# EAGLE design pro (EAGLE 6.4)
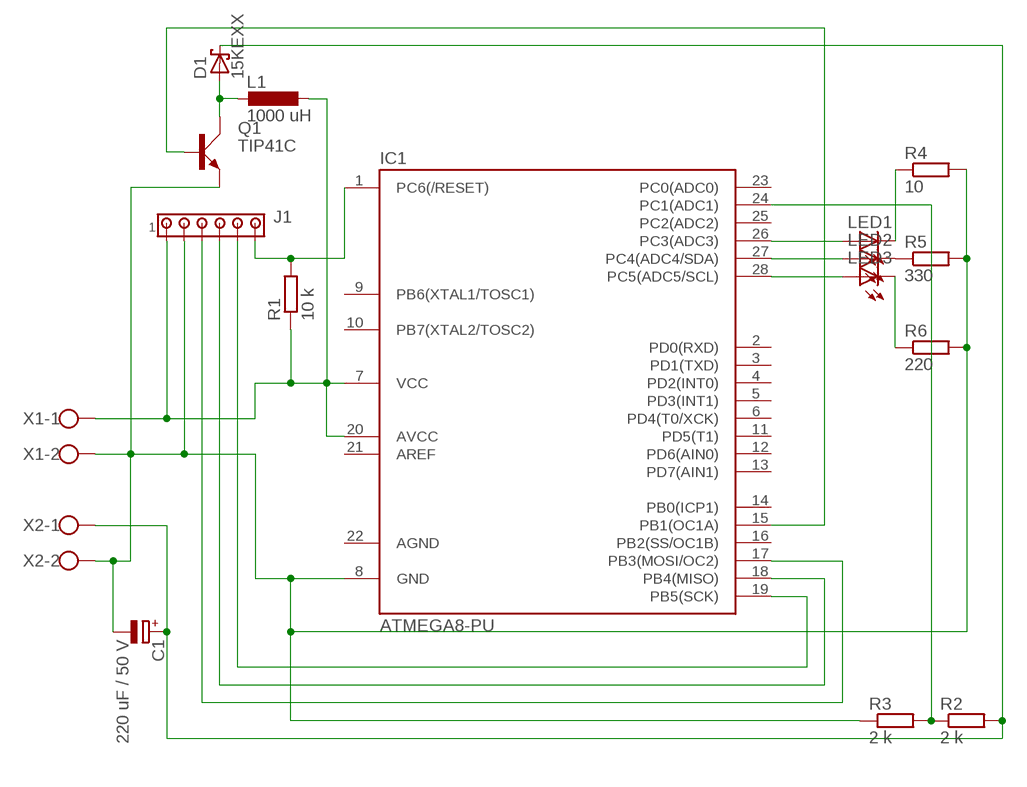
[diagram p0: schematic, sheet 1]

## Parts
C1  220 uF / 50 V  CPOL-EUE3.5-10  [E3,5-10]
D1  15KEXX  [CB429-17]
IC1  ATMEGA8-PU  [DIL28-3]
J1  MTA06-100  [10X06MTA]
L1  1000 uH  L-EUTJ5-U1  [TJ5-U1]
LED1  LED5MM  [LED5MM]
LED2  LED5MM  [LED5MM]
LED3  LED5MM  [LED5MM]
Q1  TIP41C  [TO220AV]
R1  10 k  R-EU_0204/7  [0204/7]
R2  2 k  R-EU_0204/7  [0204/7]
R3  2 k  R-EU_0204/7  [0204/7]
R4  10  R-EU_0204/7  [0204/7]
R5  330  R-EU_0204/7  [0204/7]
R6  220  R-EU_0204/7  [0204/7]
X1  W237-102  [W237-102]
X2  W237-102  [W237-102]

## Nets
N$1: IC1.7(VCC) IC1.20(AVCC) J1.6 L1.1 R1.1 X1.1
N$2: IC1.26(PC3(ADC3)) LED1.A
N$3: IC1.19(PB5(SCK)) J1.2
N$4: IC1.1(PC6(/RESET)) J1.1 R1.2
N$5: IC1.18(PB4(MISO)) J1.3
N$6: IC1.17(PB3(MOSI/OC2)) J1.4
N$7: LED1.K(C) R4.1
N$8: IC1.24(PC1(ADC1)) R2.1 R3.2
N$9: C1.+ D1.C R2.2 X2.1
N$10: D1.A L1.2 Q1.C
N$11: IC1.15(PB1(OC1A)) Q1.B
N$12: IC1.27(PC4(ADC4/SDA)) LED2.A
N$13: LED3.K(C) R6.1
N$14: LED2.K(C) R5.1
N$15: C1.- IC1.8(GND) J1.5 Q1.E R3.1 R4.2 R5.2 R6.2 X1.2 X2.2
N$16: IC1.28(PC5(ADC5/SCL)) LED3.A
Unconnected: IC1.2(PD0(RXD)) IC1.3(PD1(TXD)) IC1.4(PD2(INT0)) IC1.5(PD3(INT1)) IC1.6(PD4(T0/XCK)) IC1.9(PB6(XTAL1/TOSC1)) IC1.10(PB7(XTAL2/TOSC2)) IC1.11(PD5(T1)) IC1.12(PD6(AIN0)) IC1.13(PD7(AIN1)) IC1.14(PB0(ICP1)) IC1.16(PB2(SS/OC1B)) IC1.21(AREF) IC1.23(PC0(ADC0)) IC1.25(PC2(ADC2))

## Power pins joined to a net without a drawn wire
AGND: IC1.22(AGND)

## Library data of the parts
C1 = rcl:CPOL-EU: POLARIZED CAPACITOR, European symbol
D1 = diode:15KEXX: DIODE
IC1 = atmega8:ATMEGA8-PU
J1 = con-amp:MTA06-100: AMP connector
L1 = rcl:L-EU: INDUCTOR, European symbol
LED1-LED3 = led:LED: LED
Q1 = transistor-power:TIP41C: NPN TRANSISTOR
R1-R6 = resistor:R-EU_: RESISTOR, European symbol
X1 X2 = con-wago-500:W237-102: WAGO SCREW CLAMP; MPN: 237-102; OC_FARNELL: unknown; OC_NEWARK: 70K9898

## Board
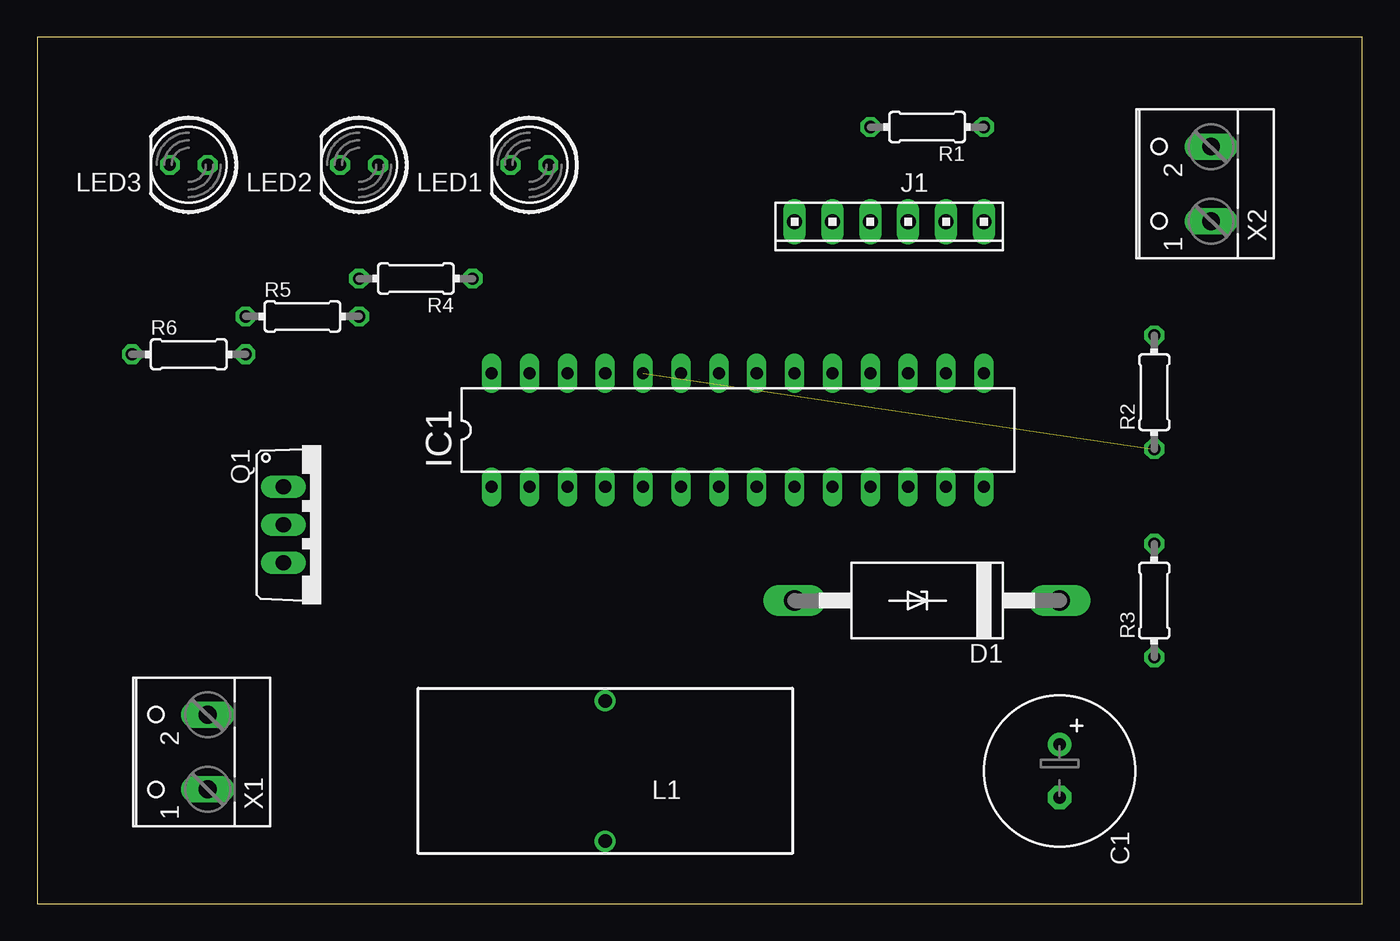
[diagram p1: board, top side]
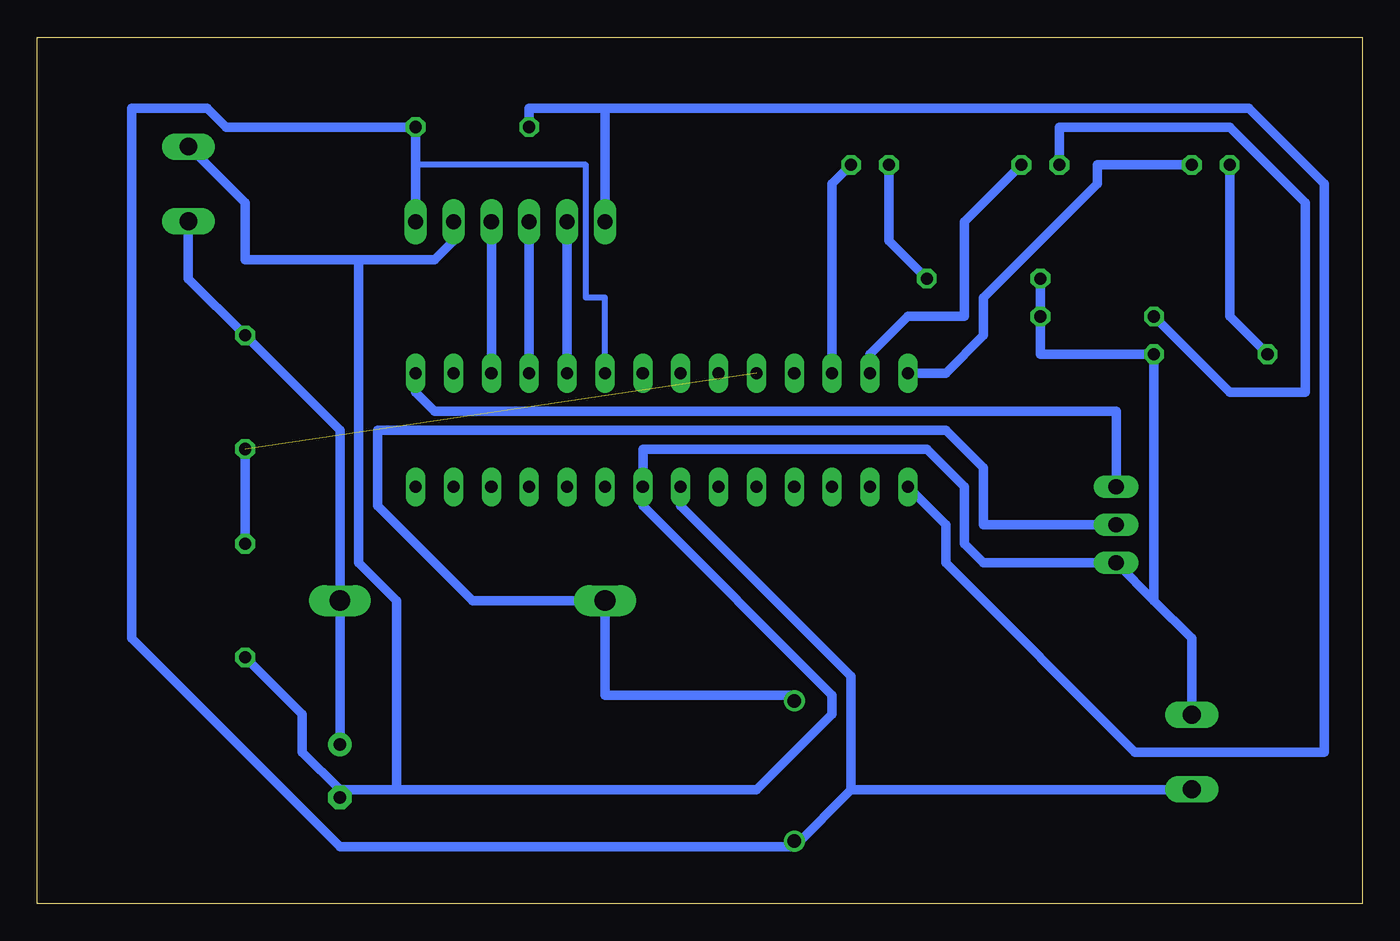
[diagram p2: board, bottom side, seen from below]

Size 88.88 x 58.09 mm. Coordinates in mm from the lower left corner, seen from the top.
Outline: 0,0 88.88,0 88.88,58.09 0,58.09 0,0
Copper layers (1*16): Top 0.035mm / dielectric 1.5mm / Bottom 0.035mm
Design rules "default *": minimum track width 25mil, minimum drill 24mil, track to track 22mil, track to pad 22mil, pad to pad 8mil, via to via 8mil, smd to smd 8mil, copper to edge 40mil, drill to drill 8mil, minimum pad ring 10mil, minimum via ring 8mil, stop-mask expansion 4mil, vias tented up to drill 0mil, thermal gap 10mil

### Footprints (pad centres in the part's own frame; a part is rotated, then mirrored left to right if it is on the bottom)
E3,5-10 = drill 0.813 pad 1.6: + -1.778,0 | drill 0.813 pad 1.6 octagon: - 1.778,0
CB429-17 = drill 1.397 long: A 8.89,0; C -8.89,0
DIL28-3 = drill 0.813 long: 1 -16.51,-3.81; 2 -13.97,-3.81; 3 -11.43,-3.81; 4 -8.89,-3.81; 5 -6.35,-3.81; 6 -3.81,-3.81; 7 -1.27,-3.81; 8 1.27,-3.81; 9 3.81,-3.81; 10 6.35,-3.81; 11 8.89,-3.81; 12 11.43,-3.81; 13 13.97,-3.81; 14 16.51,-3.81; 15 16.51,3.81; 16 13.97,3.81; 17 11.43,3.81; 18 8.89,3.81; 19 6.35,3.81; 20 3.81,3.81; 21 1.27,3.81; 22 -1.27,3.81; 23 -3.81,3.81; 24 -6.35,3.81; 25 -8.89,3.81; 26 -11.43,3.81; 27 -13.97,3.81; 28 -16.51,3.81
10X06MTA = drill 1.016 long: 1 6.35,0; 2 3.81,0; 3 1.27,0; 4 -1.27,0; 5 -3.81,0; 6 -6.35,0
TJ5-U1 = drill 0.9: 1 -4.7,0; 2 4.7,0
LED5MM = drill 0.813 octagon: A -1.27,0; K 1.27,0
TO220AV = drill 1.016 long: B -2.54,-2.54; C 0,-2.54; E 2.54,-2.54
0204/7 = drill 0.813 octagon: 1 -3.81,0; 2 3.81,0
W237-102 = drill 1.194 long: 1 -2.5,-1.27; 2 2.5,-1.27

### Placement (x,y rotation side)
C1  68.58,8.89 270 top
D1  59.69,20.32 180 top
IC1  46.99,31.75 0 top
J1  57.15,45.72 180 top
L1  38.1,8.89 90 top
LED1  33.02,49.53 180 top
LED2  21.59,49.53 180 top
LED3  10.16,49.53 180 top
Q1  19.05,25.4 270 top
R1  59.69,52.07 180 top
R2  74.93,34.29 90 top
R3  74.93,20.32 90 top
R4  25.4,41.91 180 top
R5  17.78,39.37 0 top
R6  10.16,36.83 0 top
X1  10.16,10.16 90 top
X2  77.47,48.26 90 top

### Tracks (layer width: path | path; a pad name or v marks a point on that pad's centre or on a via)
N$1
  Bottom 0.406: IC1.20 50.8,40.64 52.07,40.64 52.07,49.53 63.5,49.53
  Bottom 0.635: J1.6 63.5,49.53 R1.1 76.2,52.07 77.47,53.34 82.55,53.34 82.55,17.78 68.58,3.81 38.1,3.81 | IC1.7 45.72,26.67 34.29,15.24 34.29,7.62 | 38.1,3.81 34.29,7.62 | 34.29,7.62 11.43,7.62 X1.1 | 38.1,3.81 L1.1
N$2
  Bottom 0.635: IC1.26 35.56,48.26 LED1.A
N$3
  Bottom 0.635: J1.2 IC1.19
N$4
  Bottom 0.635: IC1.1 27.94,25.4 27.94,22.86 15.24,10.16 2.54,10.16 2.54,48.26 7.62,53.34 50.8,53.34 | 50.8,53.34 55.88,53.34 R1.2 | 50.8,53.34 J1.1
N$5
  Bottom 0.635: J1.3 IC1.18
N$6
  Bottom 0.635: J1.4 IC1.17
N$7
  Bottom 0.635: R4.1 31.75,44.45 LED1.K
N$8  (1 unrouted)
  Bottom 0.635: R2.1 R3.2
N$9
  Bottom 0.635: X2.1 78.74,41.91 R2.2 68.58,31.75 D1.C C1.+
N$10
  Bottom 0.635: L1.2 38.1,13.97 50.8,13.97 D1.A 59.69,20.32 66.04,26.67 66.04,31.75 27.94,31.75 25.4,29.21 25.4,25.4 Q1.C
N$11
  Bottom 0.635: IC1.15 63.5,34.29 62.23,33.02 16.51,33.02 Q1.B
N$12
  Bottom 0.635: IC1.27 33.02,36.83 30.48,39.37 26.67,39.37 26.67,45.72 LED2.A
N$13
  Bottom 0.635: R6.1 8.89,39.37 LED3.K
N$14
  Bottom 0.635: R5.1 8.89,34.29 3.81,34.29 3.81,46.99 8.89,52.07 20.32,52.07 LED2.K
N$15
  Bottom 0.635: R4.2 R5.2 21.59,36.83 R6.2 13.97,20.32 | 13.97,20.32 11.43,17.78 X1.2 | 13.97,20.32 Q1.E 25.4,22.86 26.67,24.13 26.67,27.94 29.21,30.48 48.26,30.48 IC1.8 48.26,26.67 35.56,13.97 35.56,12.7 40.64,7.62 64.77,7.62 | J1.5 60.96,44.45 62.23,43.18 67.31,43.18 | 67.31,43.18 74.93,43.18 74.93,46.99 78.74,50.8 X2.2 | 68.58,7.62 64.77,7.62 | R3.1 71.12,12.7 71.12,10.16 68.58,7.62 | 68.58,7.62 C1.- | 67.31,43.18 67.31,22.86 64.77,20.32 64.77,7.62
N$16
  Bottom 0.635: LED3.A 17.78,49.53 17.78,48.26 25.4,40.64 25.4,38.1 27.94,35.56 IC1.28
